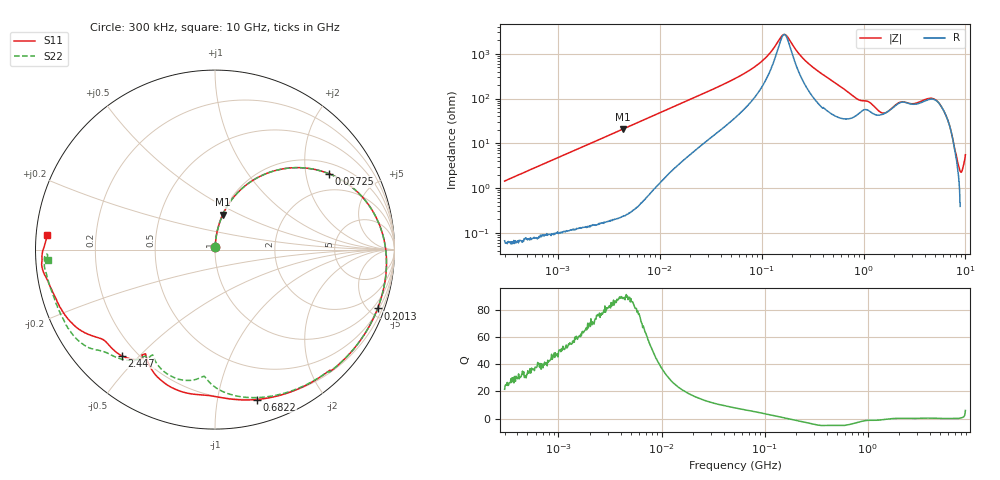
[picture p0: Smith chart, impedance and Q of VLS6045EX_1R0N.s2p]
! S-Parameter Data Generated by TDK Corporation
! Copyright(C) 2019 TDK Corporation.
! All Rights Reserved.
! TDK P/N: VLS6045EX-1R0N (Inductor)
! Property: L=1uH at 100kHz
! Size(LxWxT): 6x6x4.5mm
! Model Type: s2p (Touchstone File Format Version 1.0)
! Frequency: DC=Yes Start=0.3MHz Stop=10000MHz 802points Log-sweep
! Model Generated on May 10, 2019
! Port Assignments:
!  1 ---@@@--- 2
! Applicable Conditions:
!  Temperature = 25 degC
!  DC Bias Current = 0 A
!  Small Signal Operation
! Terms and conditions regarding TDK Simulation Models
! (1)This simulation model is being provided solely for informational purposes. Please refer to the specifications of the products in terms of detailed characteristics of such products.
! (2)In no event shall TDK Corporation of any of its subsidiaries be liable for any loss or damage arising, directly or indirectly,
!  From any information contained in this simulation model, including, but not limited to loss or damages arising from any inaccuracies, omissions or errors in connection with such information.
! (3)Any and all copyrights on this simulation model are owned by TDK Corporation.
!  Duplication or redistribution of this simulation model without prior written permission from TDK Corporation is prohibited.
! (4)This simulation model is subject to any modification or change without any prior notice.
! (5)Neither TDK Corporation nor any of its subsidiaries shall make any warranty, express or implied,
!  Including but not limited to the correctness, implied warranties of merchantability and fitness for a particular purpose with respect to this simulation models.
! (6)The use of this simulation model shall be deemed to have consented to the terms and conditions hereof.
# Hz S MA R 50
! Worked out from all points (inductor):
!   801 points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, 300 kHz to 10 GHz, reference 50 ohm
!   read as one part in series: L = 763 nH near 318.3 kHz
!   highest Q = 89 at 4.363 MHz (marker M1), where L = 759 nH
!   self-resonance near 167 MHz
!   S11 on the Smith chart (normalised r, x): 300 kHz: 1.00, +0.03; 27.25 MHz: 1.34, +2.72; 201.3 MHz: 0.61, -5.64; 682.2 MHz: 0.19, -1.30; 2.447 GHz: 0.14, -0.44; 10 GHz: 0.03, +0.04
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300000  0.01363 86.6  0.9992 -0.9  0.9993 -0.9  0.01356 86.1
1713600  0.07998 84.4  0.9954 -4.8  0.9956 -4.7  0.07999 84.3
4363314  0.2002 77.4  0.9775 -11.9  0.9775 -11.9  0.2002 77.4
9671944  0.4124 63.3  0.9004 -25.2  0.9004 -25.2  0.4123 63.3
1.694973e7  0.6112 48.0  0.7608 -39.1  0.7608 -39.1  0.6111 48.0
2.725275e7  0.7635 33.6  0.5889 -51.9  0.5889 -51.9  0.7634 33.6
5.477226e7  0.9022 14.2  0.3268 -68.1  0.3268 -68.1  0.9022 14.1
1.00316e8  0.9529 -0.8  0.1408 -75.3  0.1408 -75.3  0.9528 -0.9
1.630679e8  0.9643 -13.6  0.03566 -23.4  0.03567 -23.4  0.9642 -13.8
1.765741e8  0.9644 -15.9  0.03778 6.4  0.03778 6.4  0.9642 -16.1
2.013356e8  0.9636 -19.9  0.05922 34.1  0.05923 34.1  0.9633 -20.2
3.126428e8  0.9509 -35.7  0.1667 41.8  0.1667 41.8  0.95 -36.2
4.807079e8  0.9122 -55.1  0.2772 25.4  0.2772 25.4  0.9076 -56.3
6.821612e8  0.8673 -74.4  0.3611 4.1  0.361 4.1  0.8461 -77.0
8.528959e8  0.8273 -87.0  0.3914 -14.7  0.3914 -14.6  0.7635 -90.3
1.307877e9  0.7885 -112.2  0.3692 -43.5  0.3693 -43.5  0.7479 -108.2
1.767019e9  0.6991 -123.5  0.342 -80.7  0.342 -80.7  0.6822 -120.5
2.446702e9  0.7877 -131.4  0.18 -108.4  0.18 -108.6  0.7994 -130.1
3.34571e9  0.8115 -142.6  0.1302 -129.7  0.1296 -129.8  0.8573 -139.1
5.284132e9  0.9179 -158.7  0.04648 -142.3  0.04651 -141.7  0.9289 -153.7
7.875699e9  0.9683 -175.6  0.03311 -145.3  0.0334 -145.5  0.9551 -174.5
1e10  0.9376 174.9  0.03901 -144.0  0.03871 -143.7  0.934 -176.5
